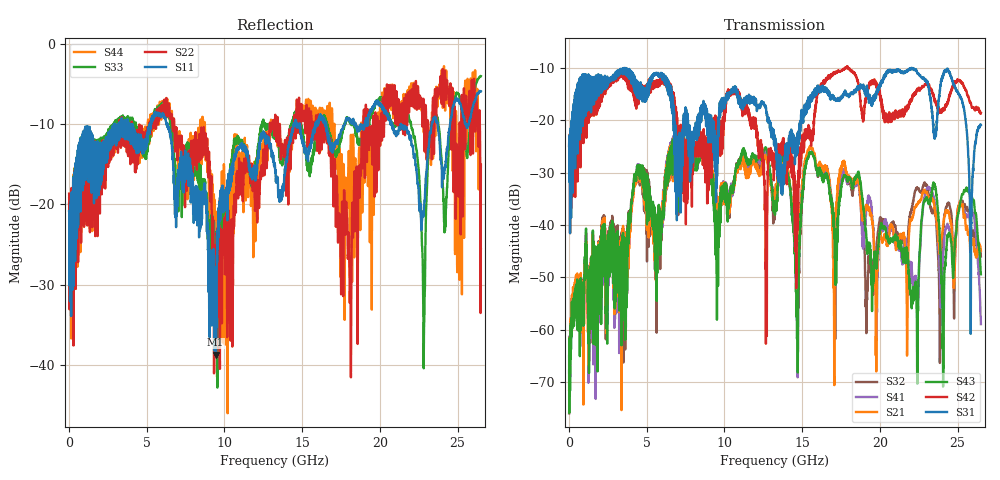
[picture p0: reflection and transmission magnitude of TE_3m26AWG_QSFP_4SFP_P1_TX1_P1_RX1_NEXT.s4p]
!Agilent Technologies,N5222A,MY51421691,A.10.00.00
!Agilent N5222A: A.10.00.00
!Date: Friday, January 30, 2015 12:33:48
!Correction: S11(Full 4 Port(1,2,3,4))
!S12(Full 4 Port(1,2,3,4))
!S13(Full 4 Port(1,2,3,4))
!S14(Full 4 Port(1,2,3,4))
!S21(Full 4 Port(1,2,3,4))
!S22(Full 4 Port(1,2,3,4))
!S23(Full 4 Port(1,2,3,4))
!S24(Full 4 Port(1,2,3,4))
!S31(Full 4 Port(1,2,3,4))
!S32(Full 4 Port(1,2,3,4))
!S33(Full 4 Port(1,2,3,4))
!S34(Full 4 Port(1,2,3,4))
!S41(Full 4 Port(1,2,3,4))
!S42(Full 4 Port(1,2,3,4))
!S43(Full 4 Port(1,2,3,4))
!S44(Full 4 Port(1,2,3,4))
!S4P File: Measurements: <S11,S12,S13,S14>,
!<S21,S22,S23,S24>,
!<S31,S32,S33,S34>,
!<S41,S42,S43,S44>:
# Hz S  dB  R 50.0
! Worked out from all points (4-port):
!   2650 points, 10 MHz to 26.5 GHz, reference 50 ohm
!   strongest paths, dB at 10 MHz, 6.63 GHz, 13.26 GHz, 19.88 GHz, 26.5 GHz:
!     S31: -24.8, -18.2, -24.4, -13.7, -20.8
!     S42: -24.9, -16.0, -29.3, -13.3, -18.6
!     S43: -67.8, -24.2, -36.5, -44.5, -49.4
!     S21: -71.5, -24.2, -34.3, -45.8, -44.9
!     S41: -65.1, -23.9, -34.9, -46.5, -58.9
!     S32: -76.0, -24.5, -35.9, -41.2, -46.0
!   lowest |S11| = -38.7 dB at 9.43 GHz (marker M1), VSWR 1.02, Z = 50.5 + j1.04 ohm
!   |S11| at or under -10 dB: start of sweep to 2.939 GHz; 6.342 GHz to 14.46 GHz (8.114 GHz wide, 78 % of centre); 21.35 GHz to 23.34 GHz (1.99 GHz wide, 8.91 % of centre)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
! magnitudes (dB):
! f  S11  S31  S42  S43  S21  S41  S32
! 10 MHz  -20.9  -24.8  -24.9  -67.8  -71.5  -65.1  -76.0
! 4.46 GHz  -12.2  -12.9  -13.8  -28.9  -28.9  -28.5  -29.2
! 9.43 GHz  -38.7  -27.4  -24.8  -37.8  -33.7  -33.4  -37.9
! 12.68 GHz  -11.9  -17.6  -45.1  -25.2  -26.7  -25.9  -26.2
! 20.11 GHz  -7.9  -12.4  -15.9  -39.7  -42.5  -40.2  -38.8
! 22.82 GHz  -21.4  -11.9  -13.5  -35.6  -33.5  -35.3  -32.5
! 26.5 GHz  -5.9  -20.8  -18.6  -49.4  -44.9  -58.9  -46.0
